TYPE ST_ToAmp8000 :
STRUCT                      				
//	FB_RUN									AT%I*	:	BOOL;
	            							
	// STATU 
	// Target System   							
	STO_Error								AT%I*	:	BOOL;
	STO_State								AT%I*	:	BOOL;
	DriveReq_Activate_Encoder				AT%I*	:	BOOL;
	DriveReq_Run							AT%I*	:	BOOL;
	DriveReq_ErrAck							AT%I*	:	BOOL;
	// Project 
	ComErr									AT%I*	:	BOOL;
	OtherErr								AT%I*	:	BOOL;
	OutErr									AT%I*	:	BOOL;
	InRun									AT%I*	:	BOOL;
	// CONTROL
	STO_ErrAct								AT%Q*	:	BOOL;
	DriveCmd_GroupErr						AT%Q*	:	BOOL;
	ErrAck									AT%Q*	:	BOOL;
	STO_Activate							AT%Q*	:	BOOL := TRUE;
END_STRUCT
END_TYPE
